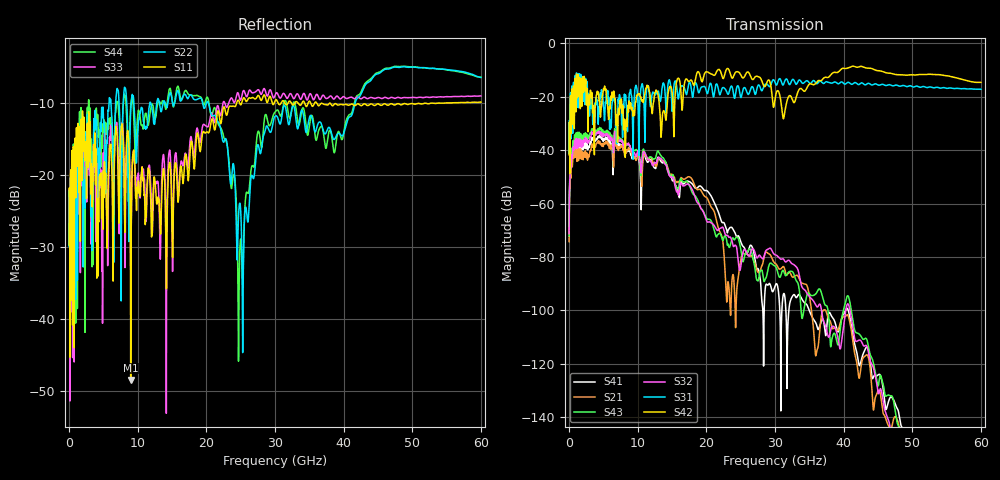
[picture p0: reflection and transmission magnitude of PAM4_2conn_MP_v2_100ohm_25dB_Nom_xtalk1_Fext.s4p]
! Info: Touchstone file created by Circ.  Input file=FAB50GbE_2conn_Midplane_Examax_Topo2_v2_100ohm_25dB_Nom.circ
# Hz S RI R 50
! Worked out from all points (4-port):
!   6000 points, 10 MHz to 60 GHz, reference 50 ohm
!   strongest paths, dB at 10 MHz, 15.01 GHz, 30.01 GHz, 45.01 GHz, 60 GHz:
!     S42: -41.7, -18.2, -20.8, -10.2, -14.6
!     S31: -41.3, -24.8, -14.5, -15.6, -17.2
!     S32: -71.2, -50.3, -79.1, -130.5, -170.6
!     S43: -72.1, -50.0, -83.3, -128.3, -170.6
!     S21: -74.2, -49.0, -82.3, -130.1, -165.6
!     S41: -69.5, -51.1, -90.9, -124.2, -168.5
!   lowest |S11| = -48.4 dB at 8.98 GHz (marker M1), VSWR 1.01, Z = 49.8 + j0.344 ohm
!   |S11| at or under -10 dB: start of sweep to 24.4 GHz; 36.9 GHz to 37.89 GHz (988.4 MHz wide, 2.64 % of centre); 38.09 GHz to 50.79 GHz (12.7 GHz wide, 28.6 % of centre)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
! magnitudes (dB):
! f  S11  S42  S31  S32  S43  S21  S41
! 10 MHz  -29.7  -41.7  -41.3  -71.2  -72.1  -74.2  -69.5
! 1.04 GHz  -14.2  -13.6  -12.7  -35.8  -33.6  -38.4  -35.2
! 8.98 GHz  -48.4  -22.3  -17.4  -39.6  -39.6  -40.6  -41.7
! 22.89 GHz  -11.6  -9.9  -17.6  -71.8  -72.9  -93.8  -69.2
! 24.87 GHz  -10.0  -11.1  -18.4  -85.0  -75.1  -83.4  -73.2
! 28.66 GHz  -9.4  -15.7  -15.2  -77.7  -88.0  -78.2  -90.5
! 60 GHz  -9.8  -14.6  -17.2  -170.6  -170.6  -165.6  -168.5
